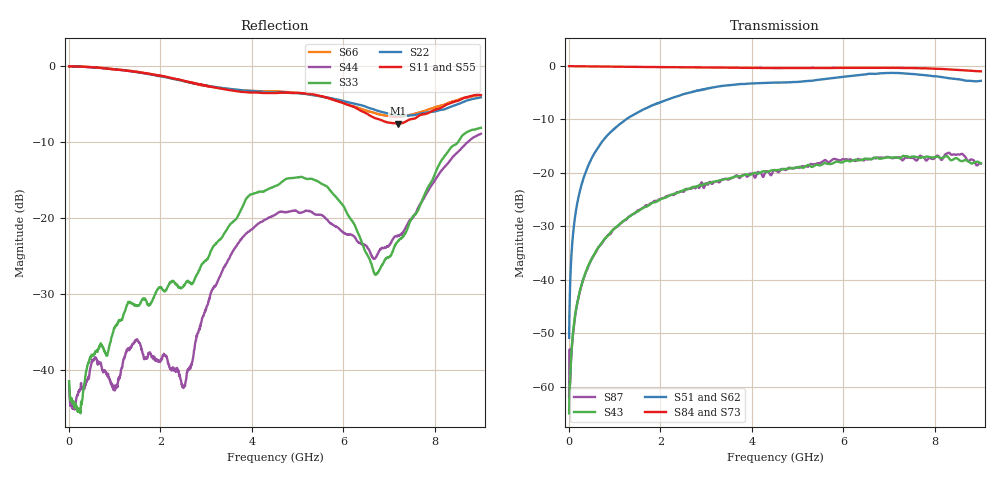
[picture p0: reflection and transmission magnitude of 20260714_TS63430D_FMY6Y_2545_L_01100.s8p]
# GHz S DB R 50
! CMT, SN0916, 25263762, 26.7.0
! Date: 15.07.2026 14:58:06
! Data: Format
! Freq S1.1:dB/Ang S1.2:dB/Ang S1.3:dB/Ang S1.4:dB/Ang S1.5:dB/Ang S1.6:dB/Ang S1.7:dB/Ang S1.8:dB/Ang
!  S2.1:dB/Ang S2.2:dB/Ang S2.3:dB/Ang S2.4:dB/Ang S2.5:dB/Ang S2.6:dB/Ang S2.7:dB/Ang S2.8:dB/Ang
!  S3.1:dB/Ang S3.2:dB/Ang S3.3:dB/Ang S3.4:dB/Ang S3.5:dB/Ang S3.6:dB/Ang S3.7:dB/Ang S3.8:dB/Ang
!  S4.1:dB/Ang S4.2:dB/Ang S4.3:dB/Ang S4.4:dB/Ang S4.5:dB/Ang S4.6:dB/Ang S4.7:dB/Ang S4.8:dB/Ang
!  S5.1:dB/Ang S5.2:dB/Ang S5.3:dB/Ang S5.4:dB/Ang S5.5:dB/Ang S5.6:dB/Ang S5.7:dB/Ang S5.8:dB/Ang
!  S6.1:dB/Ang S6.2:dB/Ang S6.3:dB/Ang S6.4:dB/Ang S6.5:dB/Ang S6.6:dB/Ang S6.7:dB/Ang S6.8:dB/Ang
!  S7.1:dB/Ang S7.2:dB/Ang S7.3:dB/Ang S7.4:dB/Ang S7.5:dB/Ang S7.6:dB/Ang S7.7:dB/Ang S7.8:dB/Ang
!  S8.1:dB/Ang S8.2:dB/Ang S8.3:dB/Ang S8.4:dB/Ang S8.5:dB/Ang S8.6:dB/Ang S8.7:dB/Ang S8.8:dB/Ang
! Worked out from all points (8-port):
!   2001 points, 10 MHz to 9 GHz, reference 50 ohm
!   strongest paths, dB at 10 MHz, 2.257 GHz, 4.505 GHz, 6.753 GHz, 9 GHz:
!     S84: -0.1, -0.3, -0.4, -0.4, -1.0
!     S73: -0.1, -0.3, -0.5, -0.5, -1.2
!     S51: -50.9, -6.0, -3.1, -1.5, -2.8
!     S62: -51.1, -6.0, -3.3, -1.8, -2.7
!     S43: -64.9, -24.1, -19.5, -17.2, -18.2
!     S87: -61.8, -24.1, -19.5, -17.2, -18.3
!   lowest |S11| = -7.6 dB at 7.184 GHz (marker M1), VSWR 2.44, Z = 21.4 - j9.42 ohm
!   |S11| at or under -10 dB: nowhere
